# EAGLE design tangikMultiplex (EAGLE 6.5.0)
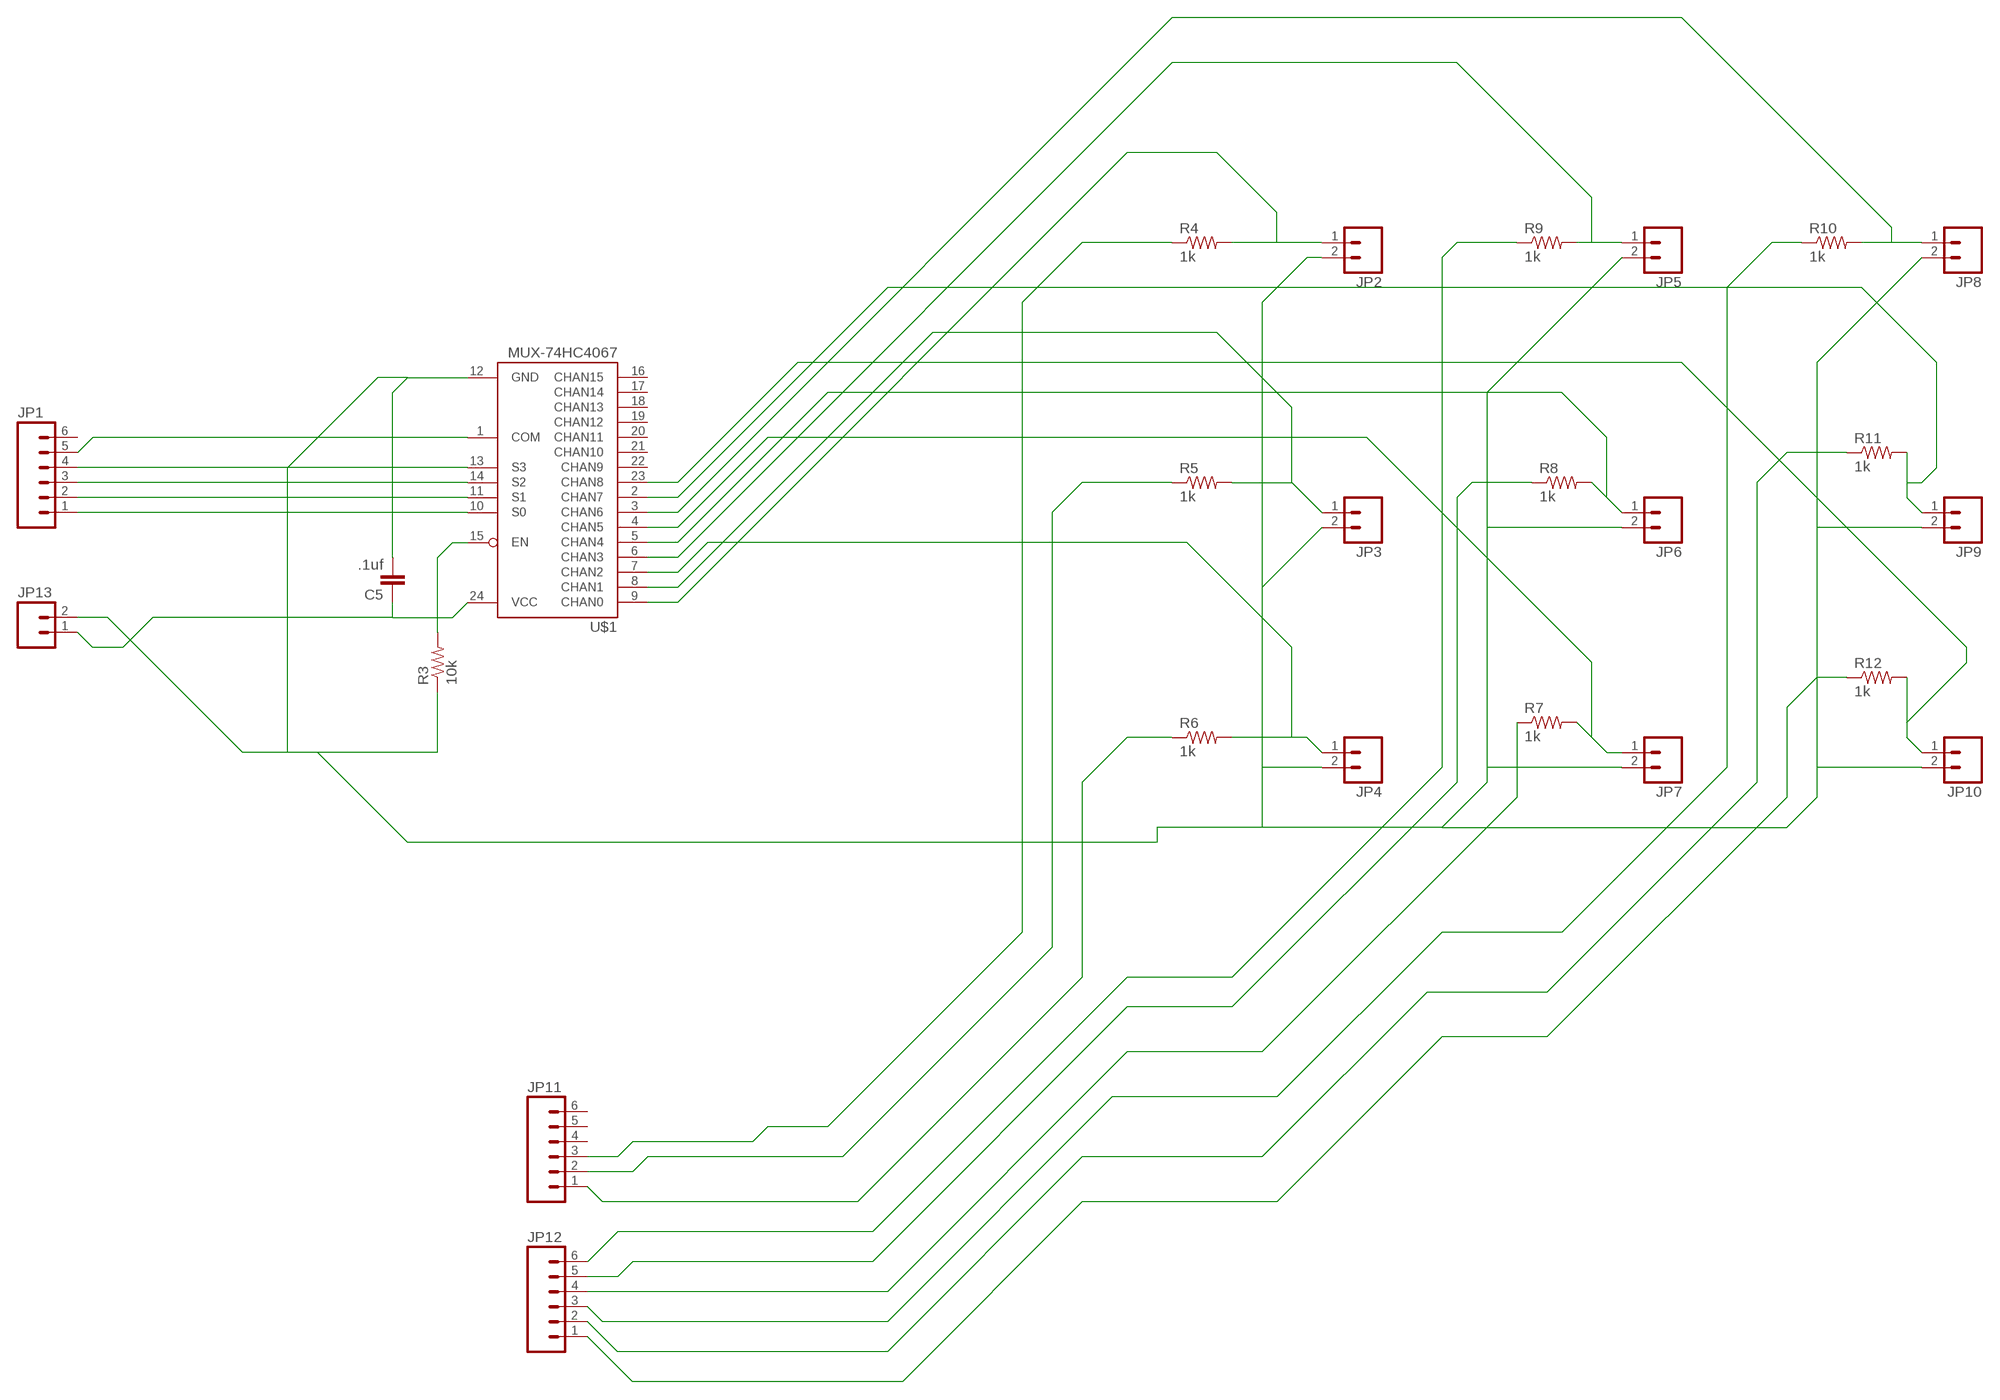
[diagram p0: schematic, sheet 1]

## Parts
C5  .1uf  C-EUC1206  [C1206]
JP1  M06LONGPADS  [1X06_LONGPADS]
JP2  M02  [1X02_LONGPADS]
JP3  M02  [1X02_LONGPADS]
JP4  M02  [1X02_LONGPADS]
JP5  M02  [1X02_LONGPADS]
JP6  M02  [1X02_LONGPADS]
JP7  M02  [1X02_LONGPADS]
JP8  M02  [1X02_LONGPADS]
JP9  M02  [1X02_LONGPADS]
JP10  M02  [1X02_LONGPADS]
JP11  M06LONGPADS  [1X06_LONGPADS]
JP12  M06LONGPADS  [1X06_LONGPADS]
JP13  M02  [1X02_LONGPADS]
R3  10k  RESISTOR1206  [1206]
R4  1k  RESISTOR1206  [1206]
R5  1k  RESISTOR1206  [1206]
R6  1k  RESISTOR1206  [1206]
R7  1k  RESISTOR1206  [1206]
R8  1k  RESISTOR1206  [1206]
R9  1k  RESISTOR1206  [1206]
R10  1k  RESISTOR1206  [1206]
R11  1k  RESISTOR1206  [1206]
R12  1k  RESISTOR1206  [1206]
U$1  MUX-74HC4067  [DIL24-6"]

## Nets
N$1: C5.1 JP13.1 U$1.24(VCC)
N$2: JP12.3 R10.1
N$4: JP10.1 R12.2 U$1.23(CHAN8)
N$5: JP1.5 U$1.1(COM)
N$7: JP1.4 U$1.13(S3)
N$8: JP11.3 R4.1
N$9: JP2.1 R4.2 U$1.9(CHAN0)
N$10: JP5.1 R9.2 U$1.6(CHAN3)
N$11: JP11.2 R5.1
N$12: JP11.1 R6.1
N$13: JP12.6 R9.1
N$14: JP12.5 R8.1
N$15: JP12.4 R7.1
N$17: JP12.2 R11.1
N$18: JP12.1 R12.1
N$21: JP9.1 R11.2 U$1.2(CHAN7)
N$22: R3.2 U$1.15(EN)
N$23: JP3.1 R5.2 U$1.8(CHAN1)
N$26: JP2.2 JP3.2 JP4.2 JP5.2 JP6.2 JP7.2 JP8.2 JP9.2 JP10.2 JP13.2 R3.1
N$29: JP4.1 R6.2 U$1.7(CHAN2)
N$30: C5.2 U$1.12(GND)
N$33: JP6.1 R8.2 U$1.5(CHAN4)
N$34: JP8.1 R10.2 U$1.3(CHAN6)
N$37: JP7.1 R7.2 U$1.4(CHAN5)
N$84: JP1.1 U$1.10(S0)
N$85: JP1.2 U$1.11(S1)
N$101: JP1.3 U$1.14(S2)
Unconnected: JP1.6 JP11.4 JP11.5 JP11.6 U$1.16(CHAN15) U$1.17(CHAN14) U$1.18(CHAN13) U$1.19(CHAN12) U$1.20(CHAN11) U$1.21(CHAN10) U$1.22(CHAN9)

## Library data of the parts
C5 = rcl:C-EU: CAPACITOR, European symbol
JP1 JP11 JP12 = 01_SparkFun:M06: Header 6 Standard 6-pin 0.1" header. Use with straight break away headers (SKU : PRT-00116), right angle break away headers (PRT-00553), swiss pins (PRT-00743), machine pins (PRT-00117), and female headers (PRT-00115). Molex polarized connector foot print use with SKU : PRT-08094 with associated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
JP2-JP10 JP13 = 01_SparkFun:M02: Header 2
R3-R12 = ng:RESISTOR
U$1 = SparkFun2:MUX-74HC4067

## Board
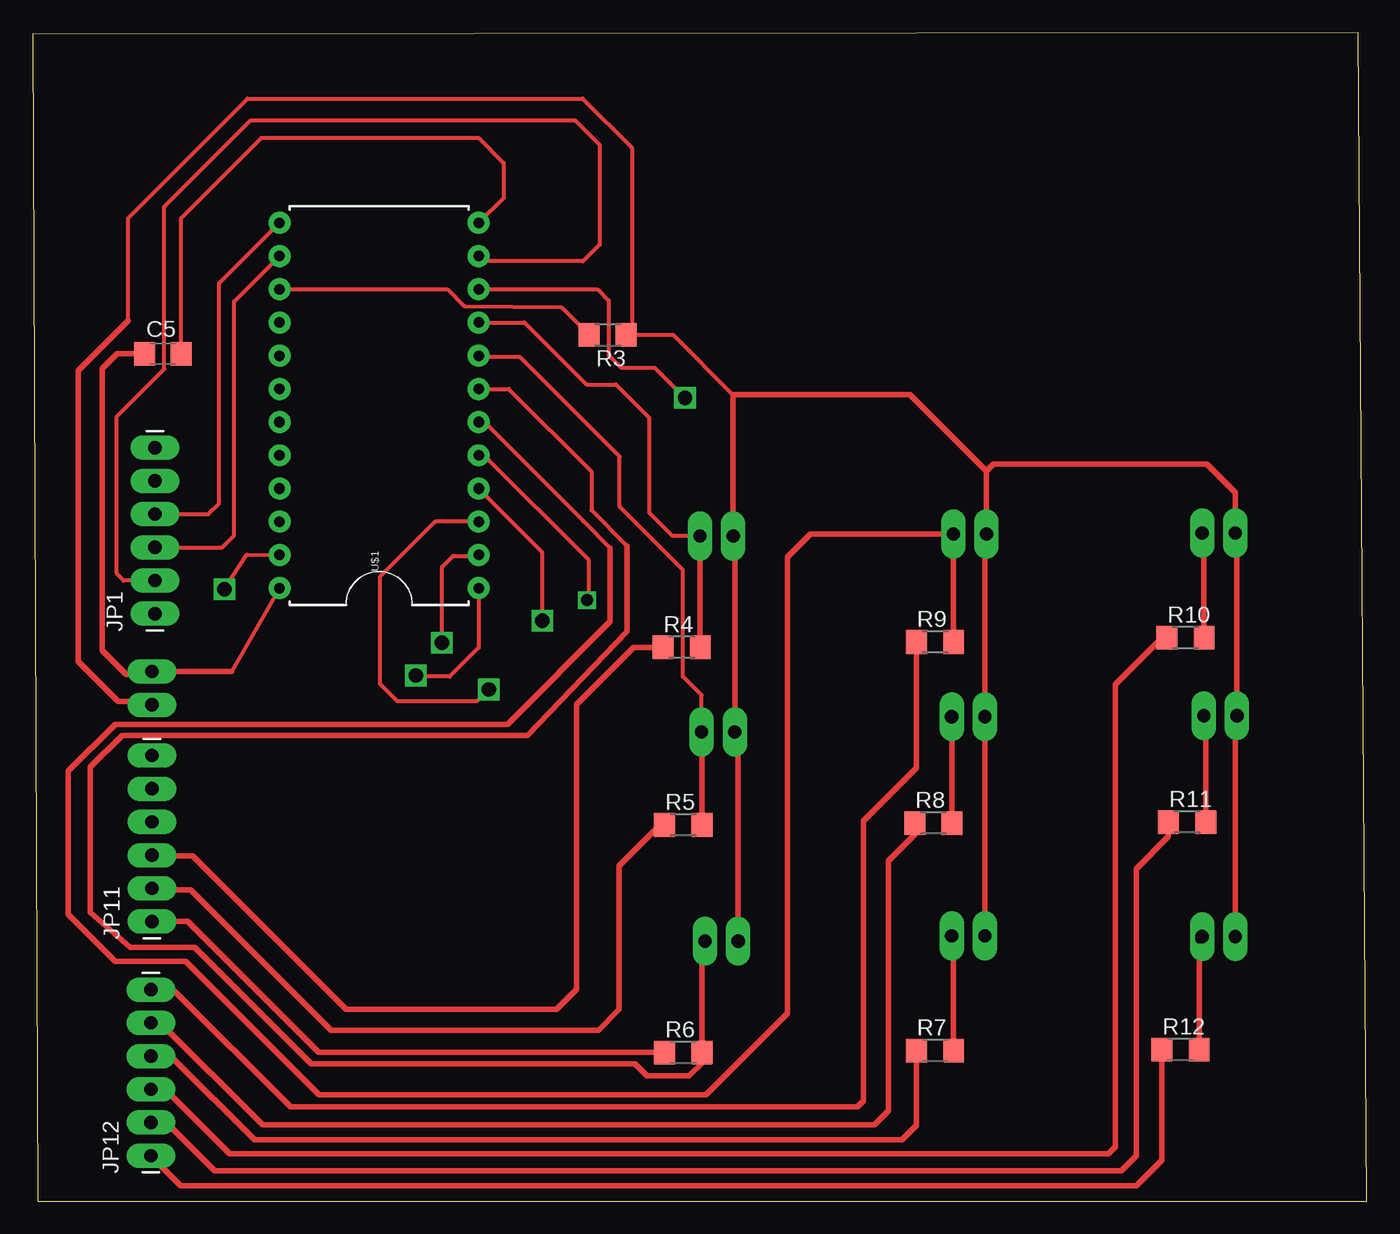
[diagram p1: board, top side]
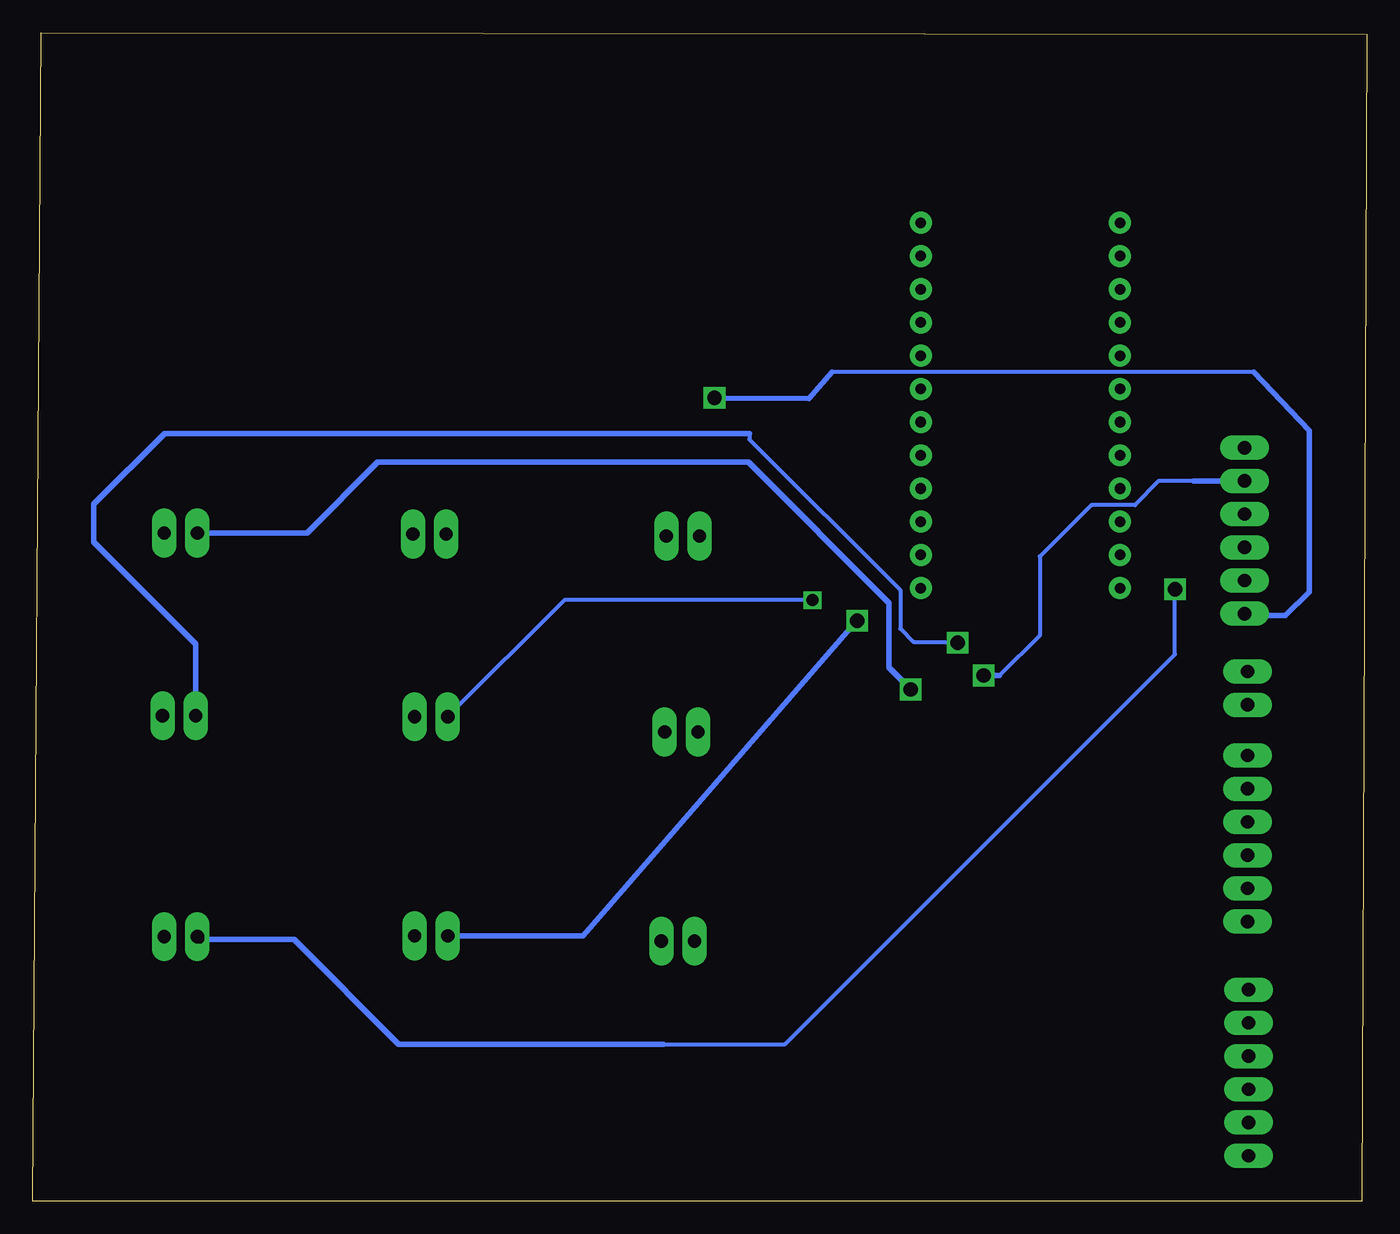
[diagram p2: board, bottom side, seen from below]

Size 102.03 x 89.37 mm. Coordinates in mm from the lower left corner, seen from the top.
Outline: 0.38,0 102.03,0 101.4,89.37 0,89.25 0.38,0
Copper layers (1*16): Top 0.035mm / dielectric 1.5mm / Bottom 0.035mm
Design rules "default": minimum track width 10mil, minimum drill 24mil, track to track 8mil, track to pad 8mil, pad to pad 8mil, via to via 8mil, smd to smd 8mil, copper to edge 40mil, drill to drill 8mil, minimum pad ring 10mil, minimum via ring 8mil, stop-mask expansion 4mil, vias tented up to drill 0mil, thermal gap 10mil

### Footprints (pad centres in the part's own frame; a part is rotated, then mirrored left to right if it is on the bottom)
C1206 = smd 1.6 x 1.8: 1 -1.4,0; 2 1.4,0
1X06_LONGPADS = drill 1.016 pad 1.88 long: 1 0,0; 2 2.54,0; 3 5.08,0; 4 7.62,0; 5 10.16,0; 6 12.7,0
1X02_LONGPADS = drill 1.016 pad 1.88 long: 1 0,0; 2 2.54,0
1206 = smd 1.6 x 1.803: 1 -1.422,0; 2 1.422,0
DIL24-6" = drill 0.813 pad 1.676: 1 -13.97,-7.62; 2 -11.43,-7.62; 3 -8.89,-7.62; 4 -6.35,-7.62; 5 -3.81,-7.62; 6 -1.27,-7.62; 7 1.27,-7.62; 8 3.81,-7.62; 9 6.35,-7.62; 10 8.89,-7.62; 11 11.43,-7.62; 12 13.97,-7.62; 13 13.97,7.62; 14 11.43,7.62; 15 8.89,7.62; 16 6.35,7.62; 17 3.81,7.62; 18 1.27,7.62; 19 -1.27,7.62; 20 -3.81,7.62; 21 -6.35,7.62; 22 -8.89,7.62; 23 -11.43,7.62; 24 -13.97,7.62

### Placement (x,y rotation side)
C5  9.96,64.82 0 top
JP1  9.35,44.93 90 top
JP2  51.03,50.88 0 top
JP3  51.16,35.89 0 top
JP4  51.41,19.89 0 top
JP5  70.41,51.03 0 top
JP6  70.28,37.06 0 top
JP7  70.28,20.29 0 top
JP8  89.43,51.1 0 top
JP9  89.56,37.13 0 top
JP10  89.43,20.24 0 top
JP11  9.12,21.39 90 top
JP12  9.04,3.48 90 top
JP13  9.12,40.51 270 top
R3  43.97,66.27 180 top
R4  49.63,42.37 0 top
R5  49.76,28.78 0 top
R6  49.76,11.38 0 top
R7  69.01,11.53 0 top
R8  68.88,28.93 0 top
R9  69.01,42.77 0 top
R10  88.16,43.1 0 top
R11  88.29,29.01 0 top
R12  87.78,11.61 0 top
U$1  26.49,60.86 90 top

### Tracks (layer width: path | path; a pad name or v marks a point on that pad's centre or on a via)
N$1
  Top 0.305: 15.23,40.51 U$1.24
  Top 0.406: C5.1 6.45,64.82 5.31,63.68 5.31,42.11 7.14,40.28 8.89,40.28 JP13.1 15.23,40.51
N$2
  Top 0.406: R10.1 86.38,43.1 82.8,39.52 82.8,4.17 82.27,3.63 15.06,3.63 10.26,8.43 9.17,8.43 JP12.3
N$3  (via drill 1.1)
  other vias: 31.29,42.72
N$4  (via drill 0.6, 1.1)
  Top 0.305: v14.66,46.81 16.38,49.45 U$1.23
  Top 0.406: R12.2 v89.2,20.02 JP10.1
  Bottom 0.305: 53.77,12.01 44.5,12.01 14.68,41.83 14.68,46.79 v14.66,46.81
  Bottom 0.406: v89.2,20.02 82.04,20.02 74.04,12.01 53.77,12.01
N$5  (via drill 0.6, 1.1)
  Top 0.305: U$1.1 34.11,42.34 31.9,40.13 29.39,40.13 v29.31,40.21
  Top 0.406: 29.39,40.28 v29.31,40.21
  Bottom 0.305: 13.23,55.07 15.95,55.07 17.73,53.24 21.06,53.24 25.02,49.33 25.02,43.28 28.09,40.21
  Bottom 0.406: v29.31,40.21 28.09,40.21 | 13.23,55.07 9.37,55.07 JP1.5
N$7
  Top 0.305: JP1.4 13.44,52.55 14.25,53.37 14.25,70.21 U$1.13
N$8
  Top 0.406: R4.1 45.95,42.37 41.58,38 41.58,16.2 40.06,14.68 23.98,14.68 12.24,26.42 9.17,26.42 JP11.3
N$9
  Top 0.305: JP2.1 48.95,50.88 47.14,52.68 47.14,59.92 44.6,62.46 42.37,62.46 37.62,67.21 U$1.9
  Top 0.406: R4.2 51.05,50.85 JP2.1
N$10
  Top 0.305: 44.17,49.96 42.15,51.98 42.08,52.05 34.54,59.59 U$1.6
  Top 0.406: R9.2 70.43,51 JP5.1 59.49,51.03 57.73,49.28 57.73,14.38 51.49,8.13 21.92,8.13 11.71,18.34 6.3,18.34 2.72,21.92 2.72,32.89 6.3,36.47 36.32,36.47 44.17,44.32 44.17,49.96
N$11
  Top 0.406: R5.1 47.98,28.78 44.86,25.65 44.86,14.68 43.26,13.08 22.84,13.08 12.09,23.82 9.22,23.82 JP11.2
N$12
  Top 0.406: JP11.1 11.86,21.39 21.87,11.38 R6.1
N$13
  Top 0.406: R9.1 67.59,33.15 63.53,29.08 63.53,7.67 63.07,7.21 19.71,7.21 10.87,16.05 9.17,16.05 JP12.6
N$14
  Top 0.406: R8.1 67.46,28.07 65.43,26.04 65.43,6.91 64.36,5.84 17.58,5.84 9.65,13.77 9.17,13.77 JP12.5
N$15
  Top 0.406: R7.1 67.59,5.79 66.5,4.7 16.97,4.7 10.72,10.95 9.2,10.95 JP12.4
N$17
  Top 0.406: R11.1 86.87,27.89 84.4,25.42 84.4,3.48 83.26,2.34 13.92,2.34 10.41,5.84 9.22,5.84 JP12.2
N$18
  Top 0.406: R12.1 86.36,3.15 84.4,1.19 11.33,1.19 JP12.1
N$21  (via drill 0.6)
  Top 0.305: v31.29,42.8 31.29,48.49 32.16,49.35 34.04,49.35 U$1.2
  Top 0.406: R11.2 89.71,36.98 JP9.1
  Bottom 0.305: 47.22,58.73 47.22,58.27 35.69,46.74 35.69,43.79 34.67,42.77 31.32,42.77 v31.29,42.8
  Bottom 0.406: JP9.1 89.56,42.62 97.36,50.42 97.36,53.32 91.95,58.73 47.22,58.73
N$22
  Top 0.305: U$1.15 31.72,69.75 33,68.48 40.44,68.38 R3.2
N$23
  Top 0.305: JP3.1 51.16,38.71 49.73,40.13 49.73,48.29 44.88,53.14 44.88,56.95 37.29,64.54 34.24,64.54 U$1.8
  Top 0.406: R5.2 51.18,35.87 JP3.1
N$26
  Top 0.305: 7.29,67.33 7.29,75.18 16.43,84.33 42.06,84.33 45.82,80.57 45.82,66.7 R3.1 48.97,66.27 53.57,61.67
  Top 0.406: JP10.2 91.97,37.01 JP9.2 92.1,50.98 JP8.2 91.97,54.2 89.81,56.36 73.46,56.36 72.95,55.86 | JP7.2 JP6.2 72.82,50.9 JP5.2 72.95,55.86 | JP4.2 53.95,35.64 JP3.2 53.7,50.75 JP2.2 53.57,61.67 53.59,61.7 67.11,61.7 72.95,55.86 | 7.29,67.33 3.48,63.53 3.48,41.28 6.53,38.23 8.86,38.23 JP13.2
N$29
  Top 0.305: 45.47,50.11 42.72,52.86 42.72,55.8 36.4,62.13 U$1.7
  Top 0.406: 51.13,19.89 JP4.1 51.18,19.66 R6.2 51.33,11.23 51.33,10.72 50.19,9.58 46.99,9.58 46.08,10.49 21.31,10.49 12.39,19.41 7.44,19.41 4.39,22.07 4.39,33.2 6.83,35.64 37.85,35.64 45.47,43.56 45.47,50.11
N$30
  Top 0.305: C5.2 11.36,75.19 17.5,81.33 34.09,81.33 36.02,79.4 36.02,76.73 U$1.12
N$33  (via drill 0.9)
  Top 0.305: U$1.5 34.52,57.05 42.49,49.07 42.49,46.08 v42.39,45.97
  Top 0.406: R8.2 70.31,37.03 JP6.1
  Bottom 0.305: v42.39,45.97 61.37,45.97 JP6.1
N$34  (via drill 0.6, 1.1)
  Top 0.305: U$1.3 30.79,51.97 26.54,47.73 26.54,39.6 27.89,38.25 33.98,38.25 v34.87,39.14
  Top 0.406: R10.2 89.58,50.95 JP8.1
  Bottom 0.406: JP8.1 81.05,51.11 75.64,56.52 47.3,56.52 36.55,45.77 36.55,40.82 v34.87,39.14
N$37  (via drill 0.6, 1.1)
  Top 0.305: v38.99,44.4 38.99,49.63 U$1.4
  Top 0.406: R7.2 70.43,20.14 JP7.1
  Bottom 0.406: JP7.1 59.94,20.29 v38.99,44.4
N$84  (via drill 1.1)
  Top 0.305: U$1.10 43.18,69.75 44.04,68.88 44.04,64.72 45.01,63.75 47.57,63.75 v49.89,61.44
  Bottom 0.305: 8.66,63.42 40.92,63.42
  Bottom 0.406: v49.89,61.44 42.65,61.39 40.92,63.42 | 8.66,63.42 4.39,58.95 4.39,46.61 6.22,44.78 9.2,44.78 JP1.1
N$85
  Top 0.305: JP1.2 6.96,47.47 6.43,48.01 6.43,60.02 10.06,63.65 10.06,76.05 16.69,82.68 41.48,82.68 43.36,80.8 43.36,73.15 42.09,71.88 34.52,71.88 U$1.11
N$101
  Top 0.305: JP1.3 14.5,50.01 15.39,50.9 15.39,68.81 U$1.14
